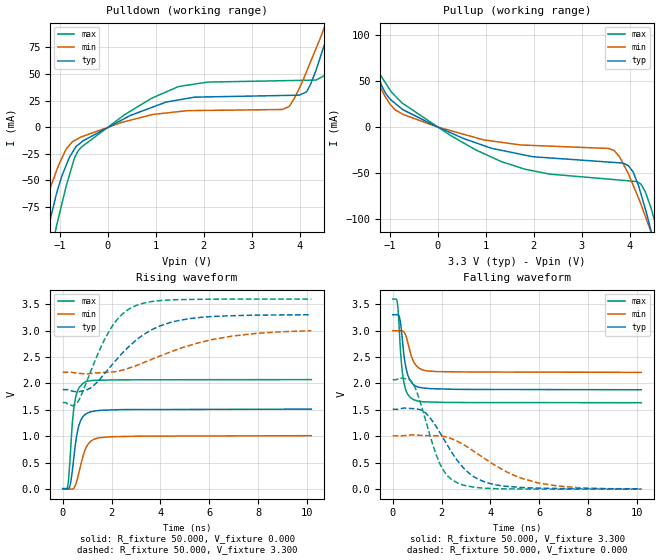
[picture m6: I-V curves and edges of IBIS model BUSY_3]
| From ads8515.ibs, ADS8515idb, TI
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|   BUSY OUTPUT Model  3V
[Model] BUSY_3
Model_type Output
Polarity   Non-Inverting
Enable   Active-Low
Vmeas = 1.65
Vref = 1.65
Cref = 15pF
Rref = 50
|   typ   min   max
|   typ   min   max
| AVERAGE
C_comp   6.6095635E-12   5.4826370E-12   7.7066390E-12
| HIGH state
|C_comp   6.9339500E-12   5.7320290E-12   7.8802020E-12
| LOW state
|C_comp   6.2851770E-12   5.2332450E-12   7.5330760E-12
[Voltage Range]   3.3   3   3.6
[Temperature Range]   27   85   -40
[Pullup Reference]   3.3   3   3.6
[Pulldown Reference]   0   0   0
[Power Clamp Reference]   3.3   3   3.6
[GND Clamp Reference]   0   0   0
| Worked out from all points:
|   slope of the pulldown table from 0 to 0.495 V, typ, clamps not added: 42 ohm
|   slope of the pullup table from 0 to 0.495 V, typ, clamps not added: 43 ohm
|   falling waveform, R_fixture 50.000, V_fixture 3.300: 20-80 % time 262ps typ, 335ps min, 209ps max; typ from 3.3 V to 1.88 V
|   rising waveform, R_fixture 50.000, V_fixture 0.000: 20-80 % time 285ps typ, 378ps min, 220ps max; typ from 0.008 V to 1.51 V
|   rising waveform, R_fixture 50.000, V_fixture 3.300: 20-80 % time 1.97ns typ, 3.05ns min, 1.25ns max; typ from 1.88 V to 3.3 V
|   falling waveform, R_fixture 50.000, V_fixture 0.000: 20-80 % time 1.37ns typ, 2.28ns min, 885ps max; typ from 1.51 V to 0.008 V
[Pulldown]
|   Voltage   I  typ   I  min   I  max
-3.3V     -573.5mA   -407.4mA   -791.3mA
-1.476V   -144.4mA   -95.47mA   -206.6mA
-1.241V   -94.58mA   -62.34mA   -135.6mA
-1.08V    -64.03mA   -42.28mA   -95.07mA
-617.8mV  -16.52mA   -10.73mA   -22.19mA
910.7mV   18.46mA    11.64mA    27.11mA
3.639V    29.75mA    16.59mA    43.64mA
4.136V    33mA       51.69mA    44.05mA
4.521V    78.62mA    94.85mA    48.91mA
4.667V    98.7mA     112.3mA    67.88mA
4.97V     143.5mA    148.8mA    122.4mA
6.59V     387.7mA    347.2mA    436.2mA
[Pullup]
|   Voltage   I  typ   I  min   I  max
-3.3V     357.5mA    294.1mA    450.1mA
-2.03V    167.1mA    139.6mA    204.5mA
-1.472V   85.35mA    73.46mA    100mA
-1.218V   51.55mA    45.91mA    58.44mA
-721.8mV  18.85mA    13.78mA    25.49mA
1.34V     -25.44mA   -16.65mA   -37.85mA
3.674V    -38.49mA   -25.44mA   -57.18mA
4.07V     -48.87mA   -63.17mA   -58.94mA
4.234V    -73.01mA   -84.32mA   -62.15mA
4.447V    -113.6mA   -114.8mA   -88.72mA
4.626V    -151.2mA   -142.4mA   -128.2mA
6.59V     -614.2mA   -486.6mA   -754.2mA
[Ramp]
R_load = 50
|   typ   min   max
dV/dt_r   0.922224/2.84181e-010   0.60547/3.73739e-010   1.24254/2.18375e-010
dV/dt_f   0.851355/2.60237e-010  0.481821/3.31684e-010   1.19615/2.07604e-010
[Falling Waveform]
R_fixture = 50.000
V_fixture = 3.300
V_fixture_min = 3.000
V_fixture_max = 3.600
C_fixture = 0.000
|  time   V  typ   V  min   V  max
0s        3.3V       2.997V     3.597V
192.4ps   3.301V     2.998V     3.521V
278.4ps   3.249V     2.999V     2.947V
353.8ps   3.017V     3V         2.4V
477.3ps   2.479V     2.963V     1.978V
634ps     2.138V     2.743V     1.782V
873.3ps   1.972V     2.398V     1.69V
1.212ns   1.917V     2.259V     1.655V
1.82ns    1.898V     2.224V     1.646V
10.18ns   1.881V     2.21V      1.636V
[Rising Waveform]
R_fixture = 50.000
V_fixture = 0.000
V_fixture_min = 0.000
V_fixture_max = 0.000
C_fixture = 0.000
|  time   V  typ   V  min   V  max
0s        7.764mV    4.963uV    1.577uV
217.1ps   4.997mV    -2.395mV   89.97mV
305ps     75.83mV    -3.367mV   603.3mV
405.8ps   393.3mV    -1.398mV   1.308V
524.5ps   857.4mV    76.33mV    1.723V
685.1ps   1.236V     350.9mV    1.928V
939.8ps   1.419V     767.2mV    2.034V
1.279ns   1.473V     941.3mV    2.058V
1.925ns   1.496V     988mV      2.064V
10.18ns   1.512V     1.009V     2.071V
[Rising Waveform]
R_fixture = 50.000
V_fixture = 3.300
V_fixture_min = 3.000
V_fixture_max = 3.600
C_fixture = 0.000
|  time   V  typ   V  min   V  max
0s        1.881V     2.21V      1.636V
594.6ps   1.837V     2.193V     1.634V
1.151ns   1.916V     2.187V     2.233V
1.917ns   2.295V     2.21V      3.002V
2.422ns   2.565V     2.25V      3.304V
2.985ns   2.812V     2.332V     3.471V
3.936ns   3.079V     2.51V      3.566V
5.218ns   3.228V     2.722V     3.589V
6.946ns   3.281V     2.896V     3.596V
10.18ns   3.3V       2.997V     3.597V
[Falling Waveform]
R_fixture = 50.000
V_fixture = 0.000
V_fixture_min = 0.000
V_fixture_max = 0.000
C_fixture = 0.000
|  time   V  typ   V  min   V  max
0s        1.512V     1.009V     2.071V
826.1ps   1.523V     1.028V     2.004V
1.349ns   1.44V      1.014V     1.301V
1.917ns   1.081V     1.007V     495.6mV
2.247ns   826.4mV    978.2mV    251mV
2.681ns   522.1mV    898.3mV    111.1mV
3.281ns   247.9mV    728.4mV    40.13mV
3.816ns   127.9mV    562.9mV    17.74mV
5.933ns   20.64mV    121mV      989.4uV
10.18ns   7.764mV    4.963uV    1.577uV
